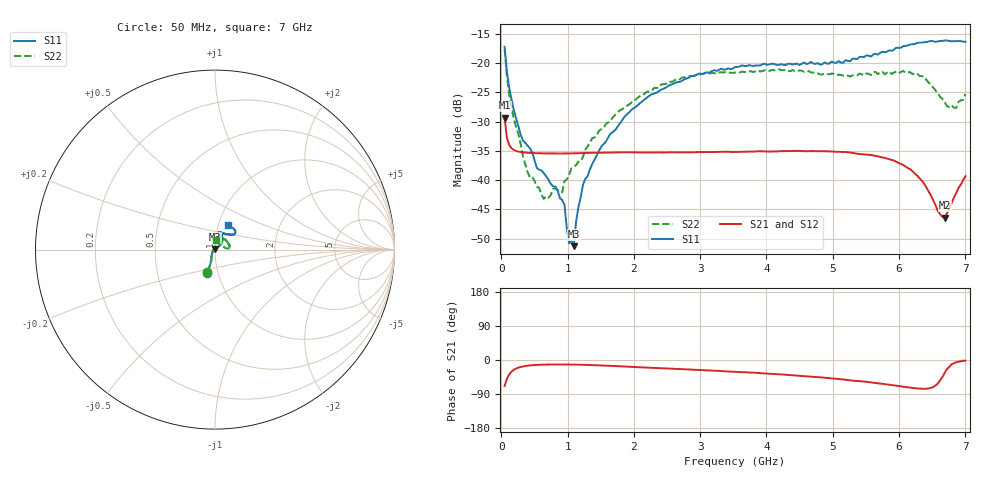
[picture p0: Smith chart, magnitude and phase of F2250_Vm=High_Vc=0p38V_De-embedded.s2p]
! Integrated Device Technology
! Corporate Headquarters
! 6024 Silver Creek Valley Road
! San Jose, CA 95138  USA
! Phone:  1-408-284-8200
! Toll Free:  1-800-223-1366
! Webpage:  http://www.idt.com/
! Timing and RF Division
! 515 Groton Road, Suite 102
! Westford, MA 01886-6024
! Device:  F2250
! Description: Voltage Variable RF Attenuator
! Frequency:  50.0 -  6000.00 MHz
! Package:  3x3 mm Thin QFN Plastic Package: 16 pin
! Ports:  2 RF, 3 DC
!  Pin  1  = GND
!  Pin  2  = NC
!  Pin  3  = RF1  = Port 1
!  Pin  4  = NC
!  Pin  5  = GND
!  Pin  6  = GND
!  Pin  7  = GND
!  Pin  8  = GND
!  Pin  9  = NC
!  Pin 10  = RF2  = Port 2
!  Pin 11  = NC
!  Pin 12  = GND
!  Pin 13  = GND
!  Pin 14  = VCNTRL
!  Pin 15  = VDD
!  Pin 16  = VMODE
! Vcntrl:  0.380 Volts
! Vmode:  +3.300 Volts
! Vdd:  +3.30  Volts
! Current:  1.261 mA
! Data:  The device was measured on a the F2250 evaluation board which has
!  individual transmission lines to the RF pins.  Data was collected
!  using a calibrated network analyzer.  The evaluation board was
!  de-embedded using a TRL calibration technique.
!  The reference plane is the edge of the package pin.
! Misc:  SN 10
!  Action Tracker AT0258
! Date Measured:  2014-11-26
! Date:  2015-10-15  MJV
! Note:
!  Integrated Device Technology supplies this data as a sample of measured
!  data at the package pin for this product.  Your particular data for this
!  product may vary.
!  Data was taken at 25 degrees C.
!  Integrated Device Technology reserves the right to change this data at anytime.
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# GHz S dB R 50
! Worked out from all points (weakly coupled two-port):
!   201 points, 50 MHz to 7 GHz, reference 50 ohm
!   highest |S21| = -29.33 dB at 50 MHz (marker M1); lowest = -46.4 dB at 6.687 GHz (marker M2)
!   lowest |S11| = -51.3 dB at 1.093 GHz (marker M3), VSWR 1.01, Z = 50 + j0.272 ohm
!   |S11| at or under -10 dB: start of sweep to end of sweep
!   |S22| runs from -43.2 to -17.6 dB; largest |S21 - S12| = 5.9e-05
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0.05  -17.17 -108.5  -29.33 -68.9  -29.33 -68.9  -17.58 -109.6
0.08475  -21.47 -107.4  -32.75 -49.5  -32.76 -49.5  -22.17 -106.6
0.189  -28.00 -119.9  -34.83 -25.9  -34.83 -25.9  -29.49 -118.5
0.328  -33.25 -134.0  -35.25 -16.9  -35.25 -16.9  -35.96 -131.3
0.43225  -34.55 -145.3  -35.35 -14.2  -35.35 -14.2  -39.53 -160.5
0.5365  -37.90 -154.6  -35.39 -12.9  -35.39 -12.9  -41.13 -176.5
0.64075  -38.80 -162.6  -35.42 -12.2  -35.42 -12.2  -43.21 153.5
0.91875  -43.43 156.1  -35.44 -11.9  -35.44 -11.9  -42.08 107.4
0.9535  -44.23 170.9  -35.44 -11.9  -35.44 -11.9  -40.17 106.5
1.023  -50.84 140.6  -35.43 -12.0  -35.43 -12.0  -39.11 88.0
1.0925  -51.30 89.6  -35.42 -12.1  -35.42 -12.1  -37.73 80.2
1.12725  -47.17 61.5  -35.40 -12.2  -35.41 -12.3  -37.46 73.0
1.2315  -40.86 40.6  -35.37 -12.6  -35.37 -12.6  -36.05 60.7
1.6485  -32.01 41.1  -35.29 -15.4  -35.29 -15.4  -29.80 52.0
2.37825  -24.76 46.7  -35.25 -21.3  -35.26 -21.3  -24.07 49.9
3.525  -20.66 71.7  -35.18 -31.0  -35.18 -31.1  -21.59 70.8
4.7065  -20.06 72.0  -35.03 -44.4  -35.03 -44.4  -21.62 69.1
5.85325  -17.79 40.5  -36.44 -65.3  -36.44 -65.3  -21.43 21.4
6.3745  -16.40 41.0  -40.55 -76.1  -40.56 -76.2  -22.24 5.1
6.68725  -16.12 47.9  -46.44 -33.9  -46.43 -33.6  -26.59 26.8
6.861  -16.21 54.5  -42.25 -6.1  -42.22 -6.0  -27.63 57.9
7  -16.32 62.4  -39.33 -1.9  -39.30 -2.0  -25.24 85.4
